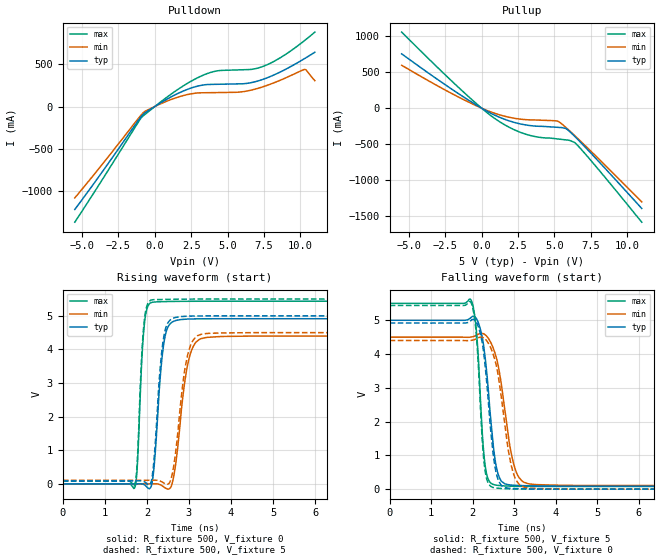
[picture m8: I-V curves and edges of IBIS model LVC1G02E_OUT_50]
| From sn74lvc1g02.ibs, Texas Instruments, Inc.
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[Model]   LVC1G02E_OUT_50
Model_type  Output
Vref =   0
Rref =   500
Cref =   50p
Vmeas =   2.5
| variable   typ   min   max
C_comp   7.96pF   5.48pF   10.59pF
| C_pullup   7.85pF   5.48pF   8.90pF
| C_pulldown   8.08pF   5.90pF   10.59pF
[Temperature Range]   40   100   -40
| Ambient temperature   25   85   -40
[Voltage range]   5   4.5   5.5
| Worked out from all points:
|   slope of the pulldown table from 0 to 0.75 V, typ, clamps not added: 9.57 ohm
|   slope of the pullup table from 0 to 0.75 V, typ, clamps not added: 9.16 ohm
|   rising waveform, R_fixture 500, V_fixture 0: 20-80 % time 174ps typ, 251ps min, 118ps max; typ from 0 V to 4.91 V
|   falling waveform, R_fixture 500, V_fixture 5: 20-80 % time 229ps typ, 322ps min, 154ps max; typ from 5 V to 0.09 V
|   rising waveform, R_fixture 500, V_fixture 5: 20-80 % time 170ps typ, 246ps min, 117ps max; typ from 0.09 V to 5 V
|   falling waveform, R_fixture 500, V_fixture 0: 20-80 % time 224ps typ, 306ps min, 152ps max; typ from 4.92 V to 0 V
[Pulldown]
| LVC1G02E_OUT_50
|   Voltage   I(typ)   I(min)   I(max)
-5.5V     -1.216A    -1.08A     -1.366A
-1.055V   -145.3mA   -124.7mA   -163.2mA
-555mV    -61.08mA   -45.82mA   -76.28mA
1.53V     149.5mA    107.5mA    195.6mA
3.15V     249mA      162mA      356.9mA
4.325V    262.7mA    164.8mA    422.2mA
5.955V    268.3mA    173.3mA    433.7mA
7.315V    314.1mA    226.7mA    466.3mA
8.65V     410.1mA    312.7mA    578.8mA
10.28V    564.5mA    437.3mA    777mA
10.41V    579.1mA    428.3mA    796.2mA
11V       641.2mA    305.2mA    879.1mA
[Pullup]
| LVC1G02E_OUT_50
|   Voltage   I(typ)   I(min)   I(max)
-5.5V     754.1mA    595.8mA    1.056A
-1.4V     176.4mA    134.9mA    252.6mA
115mV     -13.61mA   -10.17mA   -19.83mA
1.005V    -106mA     -77.72mA   -156.8mA
2.02V     -183.9mA   -130.8mA   -277.5mA
3.03V     -232mA     -158.4mA   -360.1mA
3.94V     -250.5mA   -165.2mA   -402.4mA
5.285V    -265.7mA   -186.3mA   -427.4mA
5.82V     -286.5mA   -272.8mA   -439.7mA
6.51V     -414.2mA   -401.7mA   -498.2mA
8.065V    -743.6mA   -706.8mA   -858.6mA
11V       -1.39A     -1.298A    -1.58A
[Ramp]
| LVC1G02E_OUT_50
| variable   typ   min   max
dV/dt_r   3.04/1.82E-10   2.73/2.66E-10   3.35/1.22E-10
dV/dt_f   3.02/2.43E-10   2.70/3.45E-10   3.33/1.65E-10
R_load = 500
[Rising Waveform]
| LVC1G02E_OUT_50
R_fixture =   500
C_fixture =   0
L_fixture =   0
V_fixture =   0
V_fixture_min = 0
V_fixture_max = 0
|   Time   V(typ)   V(min)   V(max)
0s        181.8pV    4.248nV    2.638nV
1.71ns    200.9uV    -14.34uV   -112.7mV
1.93ns    -19.04mV   -157.6uV   4.625V
2.135ns   118.7mV    1.916mV    5.407V
2.415ns   4.273V     -106.2mV   5.424V
2.605ns   4.818V     31.79mV    5.429V
2.78ns    4.885V     1.656V     5.432V
3.03ns    4.907V     3.857V     5.434V
3.42ns    4.914V     4.36V      5.435V
24.99ns   4.914V     4.396V     5.435V
[Falling Waveform]
| LVC1G02E_OUT_50
R_fixture =   500
C_fixture =   0
L_fixture =   0
V_fixture =   5
V_fixture_min = 4.5
V_fixture_max = 5.5
|   Time   V(typ)   V(min)   V(max)
0s        5V         4.5V       5.5V
1.96ns    5.081V     4.503V     5.599V
2.09ns    5.046V     4.559V     4.664V
2.235ns   4.463V     4.609V     1.586V
2.3ns     3.893V     4.57V      697.5mV
2.555ns   751mV      3.952V     121.6mV
2.69ns    236.7mV    3.101V     102.1mV
2.985ns   116mV      756mV      85.93mV
3.365ns   99mV       153.5mV    80.37mV
24.99ns   89.64mV    107.6mV    78.98mV
[Rising Waveform]
| LVC1G02E_OUT_50
R_fixture =   500
C_fixture =   0
L_fixture =   0
V_fixture =   5
V_fixture_min = 4.5
V_fixture_max = 5.5
|   Time   V(typ)   V(min)   V(max)
0s        89.62mV    107.6mV    78.96mV
1.705ns   89.77mV    107.6mV    -33.5mV
1.77ns    90.64mV    107.6mV    646mV
1.925ns   74.65mV    107.5mV    4.697V
2.11ns    103.7mV    109.2mV    5.474V
2.39ns    4.288V     34.94mV    5.489V
2.715ns   4.961V     1.282V     5.496V
2.975ns   4.992V     3.865V     5.499V
3.345ns   4.999V     4.467V     5.5V
24.99ns   5V         4.5V       5.5V
[Falling Waveform]
| LVC1G02E_OUT_50
R_fixture =   500
C_fixture =   0
L_fixture =   0
V_fixture =   0
V_fixture_min = 0
V_fixture_max = 0
|   Time   V(typ)   V(min)   V(max)
0s        4.917V     4.401V     5.437V
1.96ns    4.995V     4.404V     5.523V
2.085ns   4.95V      4.454V     4.589V
2.225ns   4.364V     4.497V     1.538V
2.285ns   3.823V     4.46V      670mV
2.52ns    792mV      3.889V     41.22mV
2.67ns    144.6mV    2.89V      21.03mV
2.955ns   20.8mV     574.5mV    6.836mV
3.36ns    7.024mV    29.92mV    1.3mV
24.99ns   14.81uV    18.19uV    15.7uV
